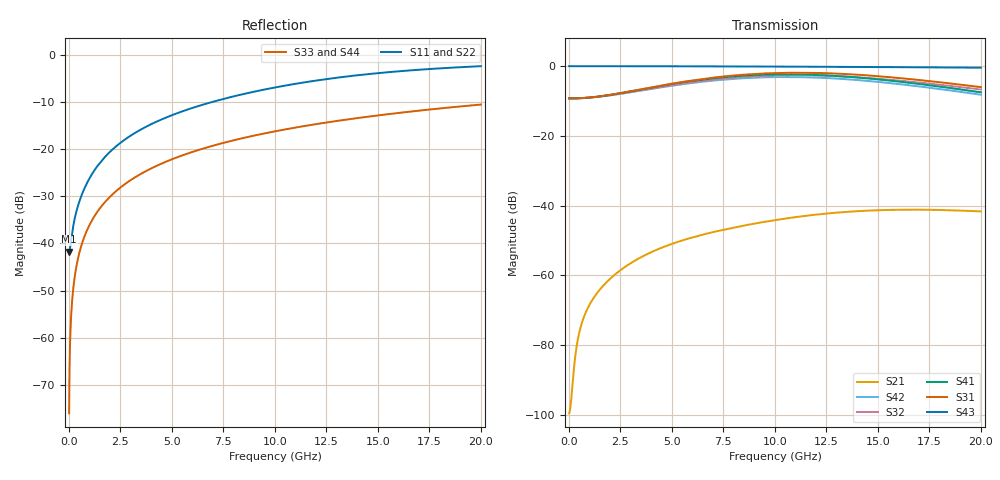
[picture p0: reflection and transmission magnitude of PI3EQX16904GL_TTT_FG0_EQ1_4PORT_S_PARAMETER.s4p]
! NPort=4 DATA=2000 NOISE=0 GROUPDELAY=0 COMPLEX_DATAFORMAT=POLAR
! NumOfBlock=1 NumOfParam=0
! .MODEL Smodel S TSTONEFILE=PI3EQX16904GL_TTT_FG0_EQ1_4PORT_S_PARAMETER.s4p TYPE=S
!  -- The above .MODEL line can be used for the S element in the netlist.
! The s parameter is extracted from the linear redriver, it is not bi-directional; only s(4,1)s(4,2) and s(3,1)s(3,2)
! should be the insertion loss
!Port definition:
!Port1 = input+
!Port2 = input-
!Port3 = output+
!Port4 = output-
# Hz S MA R  50
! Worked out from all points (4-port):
!   2000 points, 10 MHz to 20 GHz, reference 50 ohm
!   strongest paths, dB at 10 MHz, 5.01 GHz, 10.01 GHz, 15.01 GHz, 20 GHz:
!     S43: 0.0, 0.0, -0.1, -0.3, -0.4
!     S31: -9.2, -5.0, -2.0, -2.9, -6.0
!     S41: -9.2, -5.1, -2.4, -3.8, -7.5
!     S32: -9.2, -5.5, -2.7, -3.6, -6.7
!     S42: -9.2, -5.6, -3.1, -4.5, -8.2
!     S21: -99.6, -51.0, -44.2, -41.3, -41.7
!   lowest |S11| = -41.7 dB at 10 MHz (marker M1), VSWR 1.02, Z = 49.2 - j0.0603 ohm
!   |S11| at or under -10 dB: start of sweep to 6.916 GHz
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1e7  0.008182 -175.7  1.049e-05 7.4  0 0.0  0 0.0
     1.049e-05 7.4  0.008182 -175.7  0 0.0  0 0.0
     0.3451 -0.1  0.3451 179.9  0.0001571 -90.0  1 -0.0
     0.3451 179.9  0.3451 -0.1  1 -0.0  0.0001571 -90.0
2e8  0.01483 -130.6  3.32e-05 105.3  0 0.0  0 0.0
     3.32e-05 105.3  0.01483 -130.6  0 0.0  0 0.0
     0.3451 -0.1  0.345 179.7  0.003142 -90.2  1 -0.2
     0.3451 179.5  0.345 -0.7  1 -0.2  0.003142 -90.2
6.2e8  0.03268 -112.4  0.0002037 112.9  0 0.0  0 0.0
       0.0002037 112.9  0.03268 -112.4  0 0.0  0 0.0
       0.3484 -0.1  0.3478 179.2  0.009738 -90.6  0.9999 -0.6
       0.3483 178.7  0.3477 -1.9  0.9999 -0.6  0.009738 -90.6
2.97e9  0.1383 -101.7  0.001474 93.6  0 0.0  0 0.0
        0.001475 93.5  0.1383 -101.7  0 0.0  0 0.0
        0.4355 -6.9  0.4233 170.7  0.0466 -92.8  0.9988 -2.7
        0.4335 167.8  0.4214 -14.7  0.9988 -2.7  0.0466 -92.8
1.054e10  0.4762 -114.2  0.006606 38.1  0 0.0  0 0.0
          0.006539 38.1  0.4751 -114.3  0 0.0  0 0.0
          0.8035 -99.0  0.7382 80.1  0.1632 -99.8  0.9855 -9.4
          0.7613 62.7  0.6994 -118.2  0.9855 -9.4  0.1632 -99.8
1.476e10  0.6357 -124.4  0.008614 3.8  0 0.0  0 0.0
          0.008532 4.3  0.6338 -124.4  0 0.0  0 0.0
          0.7276 -160.5  0.6689 19.5  0.2254 -103.6  0.9722 -13.0
          0.6578 -5.3  0.6047 174.7  0.9722 -13.0  0.2254 -103.6
2e10  0.763 -135.6  0.008308 -33.3  0 0.0  0 0.0
      0.008267 -32.6  0.7617 -135.5  0 0.0  0 0.0
      0.5005 132.6  0.4624 -46.9  0.2986 -108.1  0.9506 -17.4
      0.4214 -79.3  0.3893 101.2  0.9506 -17.4  0.2986 -108.1
